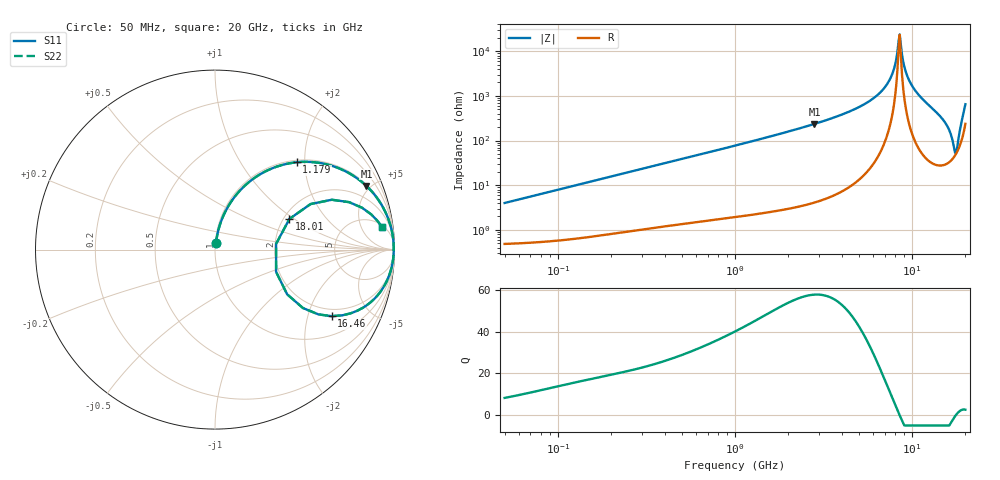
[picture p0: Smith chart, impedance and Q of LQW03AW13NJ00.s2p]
!Murata Part Number: LQW03AW13NJ00
!These Parameters are Measured in Series Mode Connection
!  o--[Z]--o
!Port1  Port2
!  o-------o
!Freq. Start=50[MHz] Stop=20[GHz], 401[Steps]
# Hz S RI R 50
!Freq.(Hz) S11(Real) S11(Imag) S21(Real) S21(Imag) S12(Real) S12(Imag) S22(Real) S22(Imag)
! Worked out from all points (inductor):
!   401 points, 50 MHz to 20 GHz, reference 50 ohm
!   read as one part in series: L = 12.6 nH near 51.52 MHz
!   highest Q = 57.7 at 2.811 GHz (marker M1), where L = 13.4 nH
!   self-resonance near 8.389 GHz
!   S11 on the Smith chart (normalised r, x): 50 MHz: 1.01, +0.08; 1.179 GHz: 1.04, +1.82; 16.46 GHz: 1.69, -2.85; 18.01 GHz: 2.15, +0.92; 20 GHz: 6, +12
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5e7  0.00638 0.0393  0.9936 -0.0393  0.9936 -0.0393  0.00638 0.0393
1.364002e8  0.0178 0.1049  0.9822 -0.1049  0.9822 -0.1049  0.0178 0.1049
3.721004e8  0.0855 0.2603  0.9145 -0.2603  0.9145 -0.2603  0.0855 0.2603
1e9  0.3756 0.4719  0.6244 -0.4719  0.6244 -0.4719  0.3756 0.4719
1.179116e9  0.4549 0.4865  0.5451 -0.4865  0.5451 -0.4865  0.4549 0.4865
2.728004e9  0.834 0.3635  0.166 -0.3635  0.166 -0.3635  0.834 0.3635
2.810964e9  0.8437 0.3546  0.1563 -0.3546  0.1563 -0.3546  0.8437 0.3546
5.433528e9  0.9745 0.1449  0.0255 -0.1449  0.0255 -0.1449  0.9745 0.1449
6.601595e9  0.9893 0.0827  0.0107 -0.0827  0.0107 -0.0827  0.9893 0.0827
7.442007e9  0.9942 0.044  0.00578 -0.044  0.00578 -0.044  0.9942 0.044
7.901521e9  0.9955 0.0243  0.00451 -0.0243  0.00451 -0.0243  0.9955 0.0243
8.264682e9  0.9959 0.00934  0.00411 -0.00934  0.00411 -0.00934  0.9959 0.00934
8.516016e9  0.9959 -0.000814  0.0041 0.000814  0.0041 0.000814  0.9959 -0.000814
8.644534e9  0.9958 -0.00594  0.00419 0.00594  0.00419 0.00594  0.9958 -0.00594
9.178299e9  0.9949 -0.0269  0.00513 0.0269  0.00513 0.0269  0.9949 -0.0269
1.004137e10  0.9914 -0.0599  0.00861 0.0599  0.00861 0.0599  0.9914 -0.0599
1.438523e10  0.9087 -0.2515  0.0913 0.2515  0.0913 0.2515  0.9087 -0.2515
1.646126e10  0.6499 -0.3708  0.3501 0.3708  0.3501 0.3708  0.6499 -0.3708
1.747767e10  0.3403 -0.124  0.6597 0.124  0.6597 0.124  0.3403 -0.124
1.800918e10  0.4147 0.1711  0.5853 -0.1711  0.5853 -0.1711  0.4147 0.1711
1.88369e10  0.7479 0.2642  0.2521 -0.2642  0.2521 -0.2642  0.7479 0.2642
2e10  0.9301 0.1258  0.0699 -0.1258  0.0699 -0.1258  0.9301 0.1258
